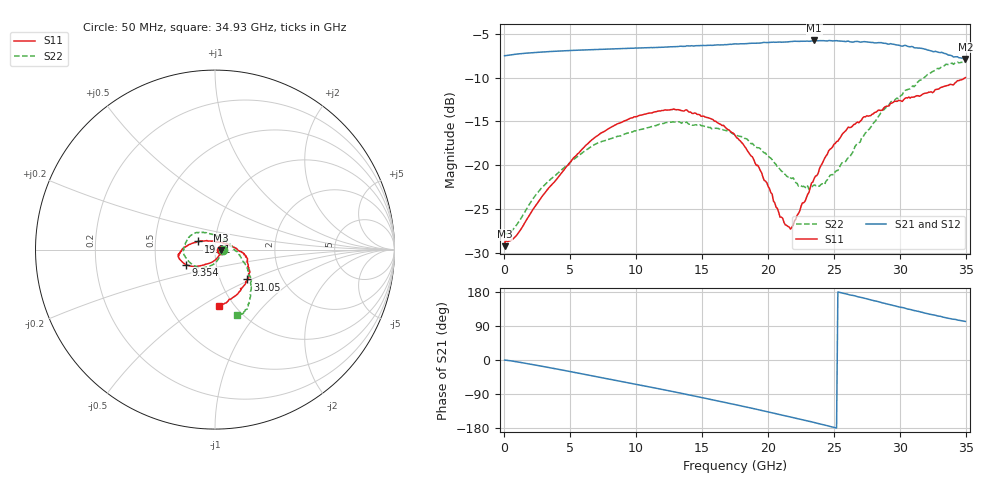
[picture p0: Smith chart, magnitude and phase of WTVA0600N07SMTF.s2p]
! 50 ohm 2-Port S-parameters measured by Modelithics Inc support@modelithics.com  Tampa, FL USA 813-866-6335 (February 2024)
! Smiths Interconnect,  6dB P/N: WTVA0600N07SMTF, Temperature: 0 C
! Board: 10 mil Rogers 4350B, Mounting Pad Dimensions: Length: 15 mils, Width: 25 mils, Gap: 40 mils.
# Hz S RI R 50
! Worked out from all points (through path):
!   352 points, 50 MHz to 34.93 GHz, reference 50 ohm
!   highest |S21| = -5.76 dB at 23.48 GHz (marker M1); lowest = -7.9 dB at 34.93 GHz (marker M2)
!   group delay of S21, straight-line fit = 21 ps
!   lowest |S11| = -29.3 dB at 50 MHz (marker M3), VSWR 1.07, Z = 53.6 - j0.194 ohm
!   |S11| at or under -10 dB: start of sweep to end of sweep
!   |S22| runs from -27.9 to -8.2 dB; largest |S21 - S12| = 0.0032
!   S11 on the Smith chart (normalised r, x): 50 MHz: 1.07, -0.00; 9.354 GHz: 0.71, -0.12; 19.01 GHz: 0.83, +0.08; 31.05 GHz: 1.34, -0.47; 34.93 GHz: 0.85, -0.60
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5e7  0.0344 -0.00181  0.4217 -0.000768  0.4215 -0.000991  0.0419 -0.00174
1e8  0.0366 -0.00456  0.4219 -0.00215  0.4218 -0.00217  0.0401 -0.0056
6.975e8  0.0281 -0.0255  0.4277 -0.0234  0.4275 -0.0234  0.0326 -0.028
2.787e9  -0.00712 -0.0643  0.425 -0.1214  0.4247 -0.1215  0.00314 -0.0731
5.8715e9  -0.0826 -0.0903  0.3668 -0.268  0.3664 -0.268  -0.0597 -0.1001
9.354e9  -0.1616 -0.0835  0.2351 -0.4006  0.2344 -0.4006  -0.1285 -0.0816
1.1742e10  -0.1968 -0.0536  0.1135 -0.4572  0.1126 -0.4572  -0.1664 -0.0401
1.38315e10  -0.2052 -0.0269  -0.00574 -0.48  -0.00609 -0.4799  -0.1759 0.00933
1.7513e10  -0.1443 0.0282  -0.2302 -0.4358  -0.2307 -0.4353  -0.1229 0.0861
1.90055e10  -0.0925 0.0452  -0.3148 -0.3851  -0.3152 -0.3846  -0.0852 0.0935
2.0299e10  -0.0457 0.0508  -0.3816 -0.3286  -0.3819 -0.328  -0.0513 0.0944
2.0896e10  -0.0208 0.046  -0.4097 -0.2948  -0.4098 -0.2943  -0.0316 0.089
2.1692e10  0.0113 0.0416  -0.4405 -0.252  -0.4406 -0.2514  -0.00871 0.0839
2.2289e10  0.0357 0.0391  -0.4615 -0.2132  -0.4619 -0.2121  0.0111 0.0752
2.33835e10  0.0751 0.0277  -0.4933 -0.1418  -0.4932 -0.1412  0.0423 0.0633
2.3483e10  0.0798 0.026  -0.4977 -0.134  -0.4976 -0.1334  0.0465 0.0615
2.4279e10  0.109 0.012  -0.5081 -0.072  -0.508 -0.0713  0.066 0.0412
2.607e10  0.1631 -0.0239  -0.5073 0.0629  -0.5069 0.0635  0.1104 -0.00252
2.91545e10  0.1882 -0.1102  -0.4107 0.2689  -0.4099 0.2696  0.187 -0.1199
3.1045e10  0.1798 -0.1663  -0.3048 0.3559  -0.303 0.3571  0.1944 -0.202
3.3433e10  0.105 -0.2631  -0.1578 0.4037  -0.1573 0.4036  0.1816 -0.3299
3.49255e10  0.0211 -0.3154  -0.0827 0.3958  -0.0805 0.396  0.1223 -0.3665
